(* Logix 5000 AddOnInstructionDefinition export Banner_VSM_Param_v4; software revision 33.00 *)

TYPE Banner_IOL_Port_v4 :   // UDT that has all of the data items necessary to communicate with a specific Port on a IO-Link Master
STRUCT
   Port_Controlled : INT;   // Each bit represents a port on an IO-Link Master. Set to 1 to tell AOI to control that port.
   Port_Activate : INT;   // Each bit represents a port on an IO-Link Master. When ON that port will process any commands in queue.
   Port_Read : INT;   // Each bit represents a port on an IO-Link Master. Used to determine when device AOI has requested a Read command.
   Port_Write : INT;   // Each bit represents a port on an IO-Link Master. Used to determine when device AOI has requested a Write command.
   Port_RW_Complete : INT;   // Each bit represents a port on an IO-Link Master. Tells device AOI that Read or Write request has been completed.
   Port_Device_Read : INT;
   Data_Transfer : SINT[190];   // Array to transfer data from IO-Master to device AOIs.
END_STRUCT
END_TYPE

TYPE Banner_VSM_RD_v4 :   // UDT that stores the Read Data for a VSM-2.
STRUCT
   Master_Cycle_Time : INT;
   Min_Cycle_Time : INT;
   Frame_Capability : INT;
   IO_Link_Version_ID : INT;
   Process_Data_Input_Length : INT;
   Process_Data_Output_Length : INT;
   Combined_Vendor_ID : DINT;   // IO-Link Vendor ID
   Vendor_ID1 : INT;
   Vendor_ID2 : INT;
   Combined_Device_ID : DINT;   // IO-Link Device ID
   Device_ID1 : INT;
   Device_ID2 : INT;
   Device_ID3 : INT;
   Maximum_Temp : INT;
   Actual_Temp : INT;
END_STRUCT
END_TYPE

TYPE Banner_VSM_v4 :   // All of the parameters for a VSM-2.
STRUCT
   Initial_Global_Read : BOOL;   // Determines if all of the IO-Link data has been read into the PLC yet
   Command : INT;   // Value placed in here will activate a read or write to a specifc IO-Link Index
   Read : Banner_VSM_RD_v4;   // Read Only Data
   Write : Banner_VSM_WD_v4;   // Write Data
   Archive : Banner_VSM_WD_v4;   // Archive Data
   Reset : BOOL;   // Resets AOI. This will force a complete parameter read of the sensor.
END_STRUCT
END_TYPE

TYPE Banner_VSM_WD_v4 :   // UDT that stores the Write Data for a VSM-2.
STRUCT
   Switching_Delay_TB : SINT;   // 0 = .1ms, 1 = .4ms, 2 = 1.6ms, 3 = 6.4ms.
   Output_Stretch_TB : SINT;   // 0 = .1ms, 1 = .4ms, 2 = 1.6ms, 3 = 6.4ms.
   Output_1_Config : SINT;   // 0 = Detection light on, 1 = Dection dark on, 2 = Stability alarm, 3 = Stability alarm inverted.
   Output_2_Config : SINT;   // 0 = Detection light on, 1 = Dection dark on, 2 = Stability alarm, 3 = Stability alarm inverted.
   Swtiching_Delay_Multiplier : INT;   // 0 to 255.
   Output_Stretch_Multiplier : INT;   // 0 to 255.
   Sensitivity : INT;   // 0 to 1023.
   Sequence_Choice : SINT;   // 0 to 9.
   Sensor_Mode : SINT;   // 1 = Fine, 2 = Normal, 3 = Fast.
   Teach_Command : SINT;   // 0 = Idle, 1 = Teach 1 Pt, 2 = Teach 2 Pt on target, 3 = Teach 2 Pt without target.
   Detection_Counter : DINT;   // 0 to 65535.
   Event_Flag_LED_Reg_Limit : SINT;
   Event_Flag_Disturbance_On_Receiver : SINT;
   Event_Flag_Under_Voltage_IOL : SINT;
   Event_Flag_Under_Voltage_Sensor : SINT;
   Event_Flag_Maximum_Temp : SINT;
   Event_Flag_EMC_Detected : SINT;
   Event_Flag_Short_Circuit_Detected : SINT;
END_STRUCT
END_TYPE

ADD_ON_INSTRUCTION Banner_VSM_Param_v4   (* revision 4.0, vendor Banner Engineering *)
// AOI to read and write parameter data to an IO-Link VSM-2.
VAR_IN_OUT
   VSM : Banner_VSM_v4; {required}
   Port_Data : Banner_IOL_Port_v4; {required}
END_VAR
VAR_INPUT
   Port : DINT; {required}
END_VAR
VAR
   Local_Control : DINT; {access None}
   Global_Read_Command_Value : INT; {access None}
   Global_Write_Command_Value : INT; {access None}
   Command_Being_Processed : BOOL; {access None}
   Update_Archive : BOOL; {access None}
   Index_Write_Inprocess : INT; {access None}
   Index_Write_Control : INT; {access None}
   Inprocess_Index : DINT; {access None}
END_VAR

ROUTINE Logic   (* ladder *)
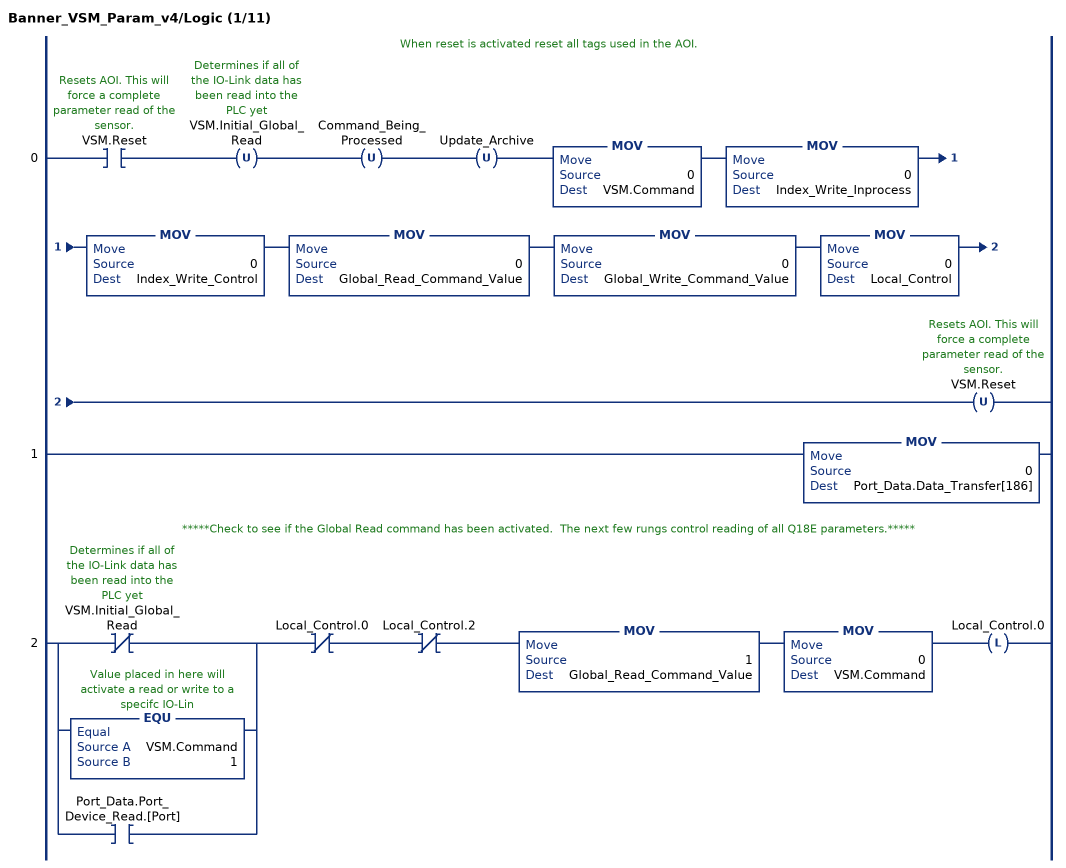
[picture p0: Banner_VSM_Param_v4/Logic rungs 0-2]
   // When reset is activated reset all tags used in the AOI.
   0: XIC(VSM.Reset)OTU(VSM.Initial_Global_Read)OTU(Command_Being_Processed)OTU(Update_Archive)MOV(0,VSM.Command)MOV(0,Index_Write_Inprocess)MOV(0,Index_Write_Control)MOV(0,Global_Read_Command_Value)MOV(0,Global_Write_Command_Value)MOV(0,Local_Control)OTU(VSM.Reset);
   1: MOV(0,Port_Data.Data_Transfer[186]);
   // *****Check to see if the Global Read command has been activated.  The next few rungs control reading of all Q18E parameters.*****
   2: [XIO(VSM.Initial_Global_Read) ,EQU(VSM.Command,1) ,XIC(Port_Data.Port_Device_Read.[Port]) ]XIO(Local_Control.0)XIO(Local_Control.2)MOV(1,Global_Read_Command_Value)MOV(0,VSM.Command)OTL(Local_Control.0);
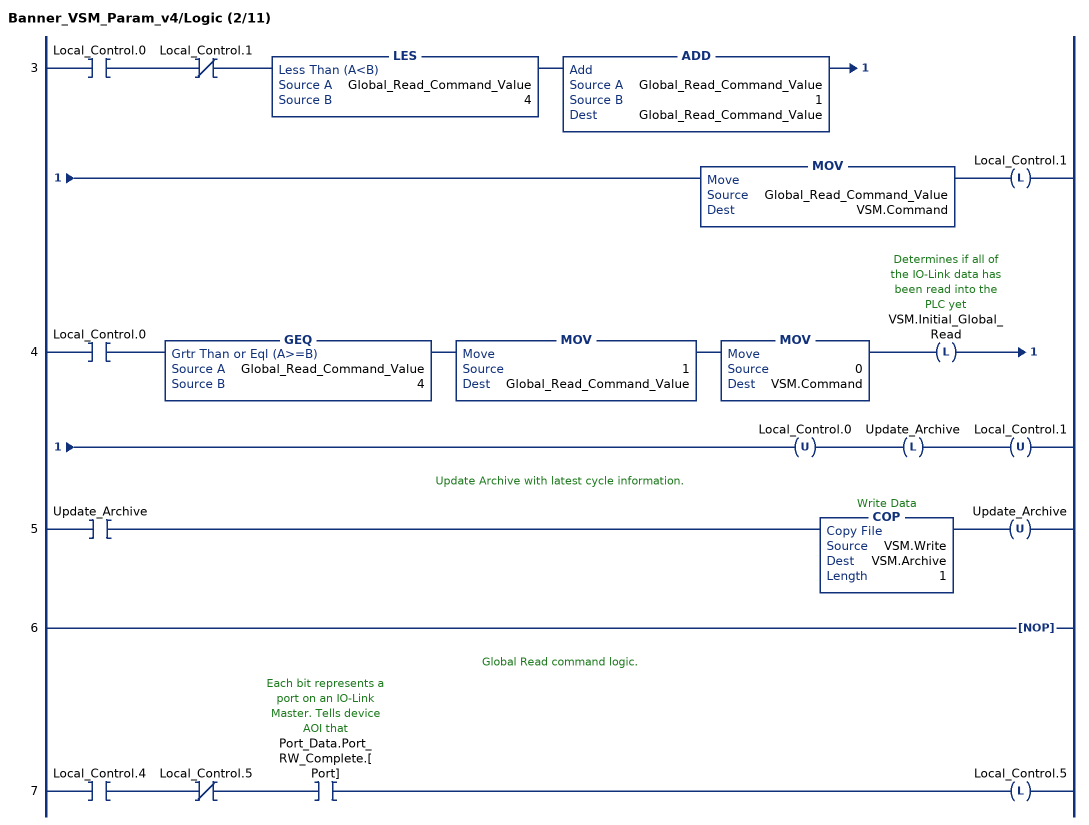
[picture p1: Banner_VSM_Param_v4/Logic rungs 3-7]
   3: XIC(Local_Control.0)XIO(Local_Control.1)LES(Global_Read_Command_Value,4)ADD(Global_Read_Command_Value,1,Global_Read_Command_Value)MOV(Global_Read_Command_Value,VSM.Command)OTL(Local_Control.1);
   4: XIC(Local_Control.0)GEQ(Global_Read_Command_Value,4)MOV(1,Global_Read_Command_Value)MOV(0,VSM.Command)OTL(VSM.Initial_Global_Read)OTU(Local_Control.0)OTL(Update_Archive)OTU(Local_Control.1);
   // Update Archive with latest cycle information.
   5: XIC(Update_Archive)COP(VSM.Write,VSM.Archive,1)OTU(Update_Archive);
   6: NOP();
   // Global Read command logic.
   7: XIC(Local_Control.4)XIO(Local_Control.5)XIC(Port_Data.Port_RW_Complete.[Port])OTL(Local_Control.5);
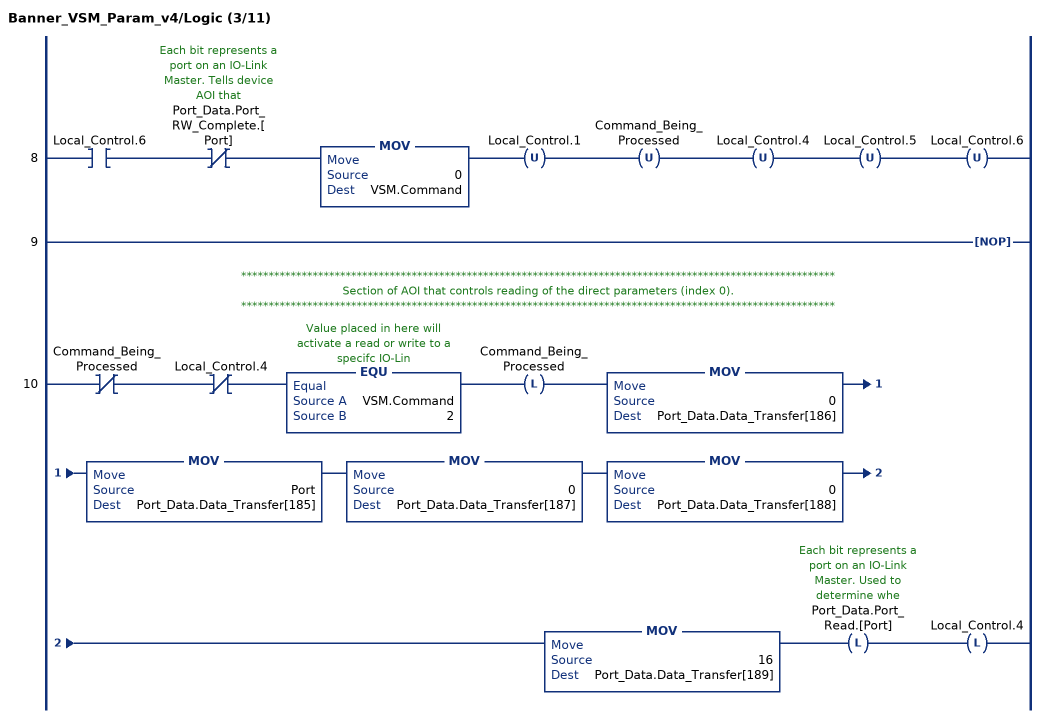
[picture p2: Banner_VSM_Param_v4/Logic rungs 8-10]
   8: XIC(Local_Control.6)XIO(Port_Data.Port_RW_Complete.[Port])MOV(0,VSM.Command)OTU(Local_Control.1)OTU(Command_Being_Processed)OTU(Local_Control.4)OTU(Local_Control.5)OTU(Local_Control.6);
   9: NOP();
   // ************************************************************************************************************
   // Section of AOI that controls reading of the direct parameters (index 0).
   // ************************************************************************************************************
   10: XIO(Command_Being_Processed)XIO(Local_Control.4)EQU(VSM.Command,2)OTL(Command_Being_Processed)MOV(0,Port_Data.Data_Transfer[186])MOV(Port,Port_Data.Data_Transfer[185])MOV(0,Port_Data.Data_Transfer[187])MOV(0,Port_Data.Data_Transfer[188])MOV(16,Port_Data.Data_Transfer[189])OTL(Port_Data.Port_Read.[Port])OTL(Local_Control.4);
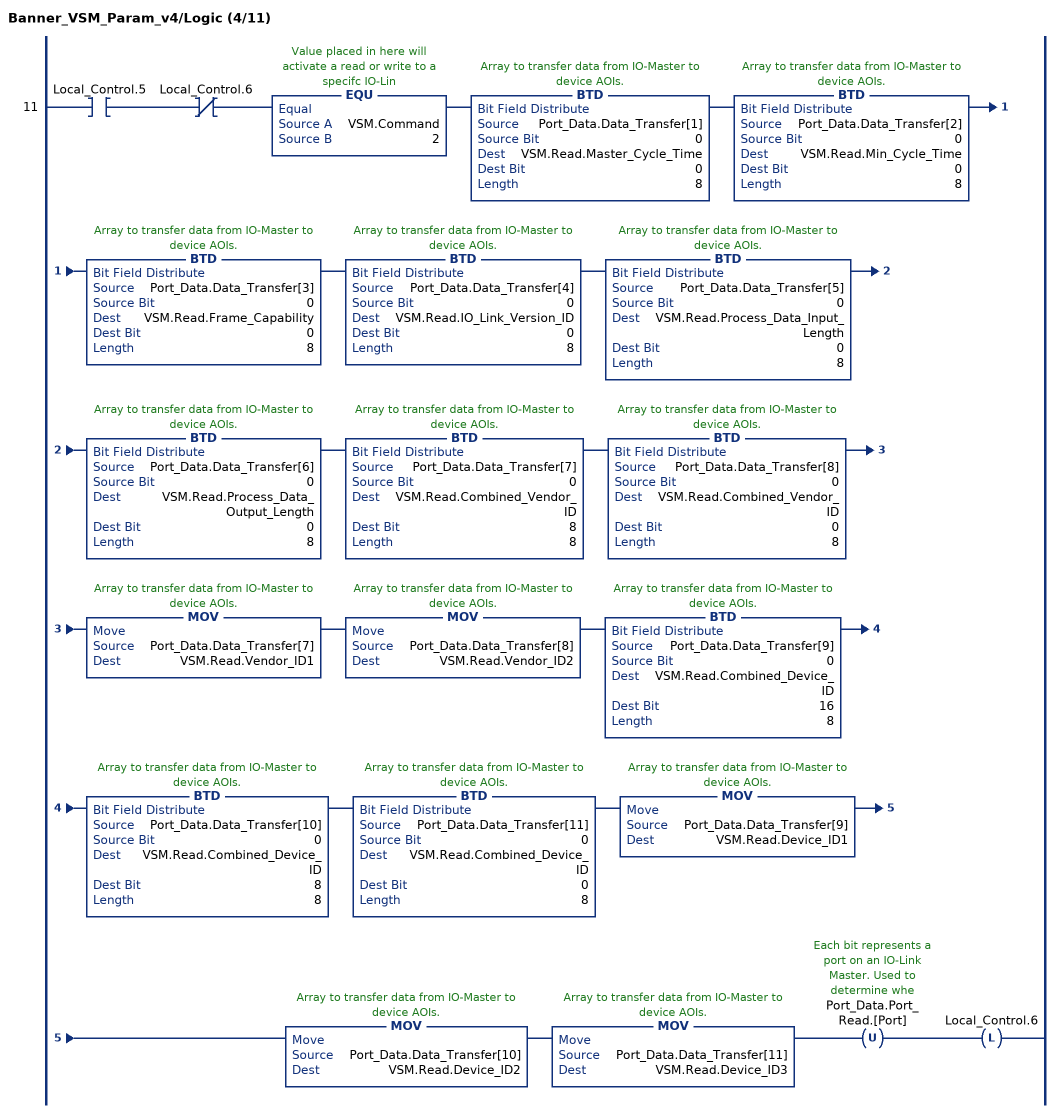
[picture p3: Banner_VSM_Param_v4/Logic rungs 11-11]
   11: XIC(Local_Control.5)XIO(Local_Control.6)EQU(VSM.Command,2)BTD(Port_Data.Data_Transfer[1],0,VSM.Read.Master_Cycle_Time,0,8)BTD(Port_Data.Data_Transfer[2],0,VSM.Read.Min_Cycle_Time,0,8)BTD(Port_Data.Data_Transfer[3],0,VSM.Read.Frame_Capability,0,8)BTD(Port_Data.Data_Transfer[4],0,VSM.Read.IO_Link_Version_ID,0,8)BTD(Port_Data.Data_Transfer[5],0,VSM.Read.Process_Data_Input_Length,0,8)BTD(Port_Data.Data_Transfer[6],0,VSM.Read.Process_Data_Output_Length,0,8)BTD(Port_Data.Data_Transfer[7],0,VSM.Read.Combined_Vendor_ID,8,8)BTD(Port_Data.Data_Transfer[8],0,VSM.Read.Combined_Vendor_ID,0,8)MOV(Port_Data.Data_Transfer[7],VSM.Read.Vendor_ID1)MOV(Port_Data.Data_Transfer[8],VSM.Read.Vendor_ID2)BTD(Port_Data.Data_Transfer[9],0,VSM.Read.Combined_Device_ID,16,8)BTD(Port_Data.Data_Transfer[10],0,VSM.Read.Combined_Device_ID,8,8)BTD(Port_Data.Data_Transfer[11],0,VSM.Read.Combined_Device_ID,0,8)MOV(Port_Data.Data_Transfer[9],VSM.Read.Device_ID1)MOV(Port_Data.Data_Transfer[10],VSM.Read.Device_ID2)MOV(Port_Data.Data_Transfer[11],VSM.Read.Device_ID3)OTU(Port_Data.Port_Read.[Port])OTL(Local_Control.6);
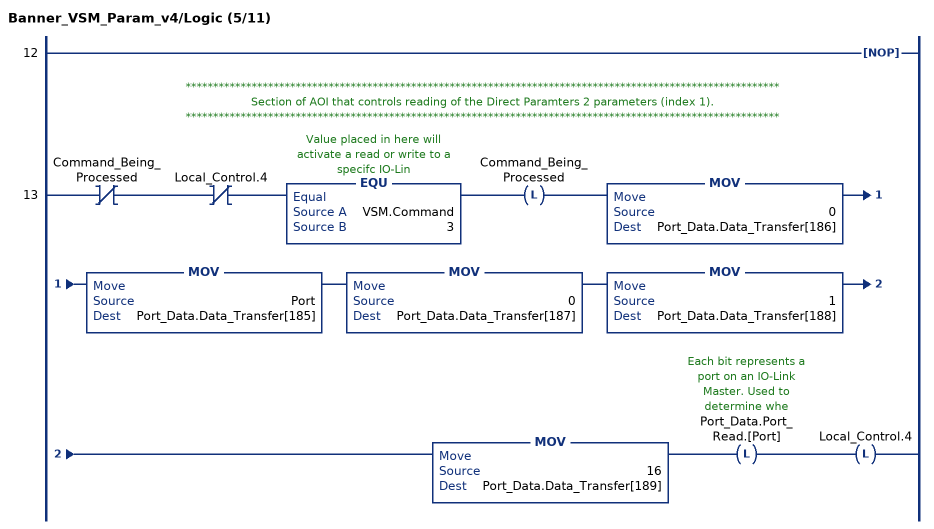
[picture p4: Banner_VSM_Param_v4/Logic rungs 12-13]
   12: NOP();
   // ************************************************************************************************************
   // Section of AOI that controls reading of the Direct Paramters 2 parameters (index 1).
   // ************************************************************************************************************
   13: XIO(Command_Being_Processed)XIO(Local_Control.4)EQU(VSM.Command,3)OTL(Command_Being_Processed)MOV(0,Port_Data.Data_Transfer[186])MOV(Port,Port_Data.Data_Transfer[185])MOV(0,Port_Data.Data_Transfer[187])MOV(1,Port_Data.Data_Transfer[188])MOV(16,Port_Data.Data_Transfer[189])OTL(Port_Data.Port_Read.[Port])OTL(Local_Control.4);
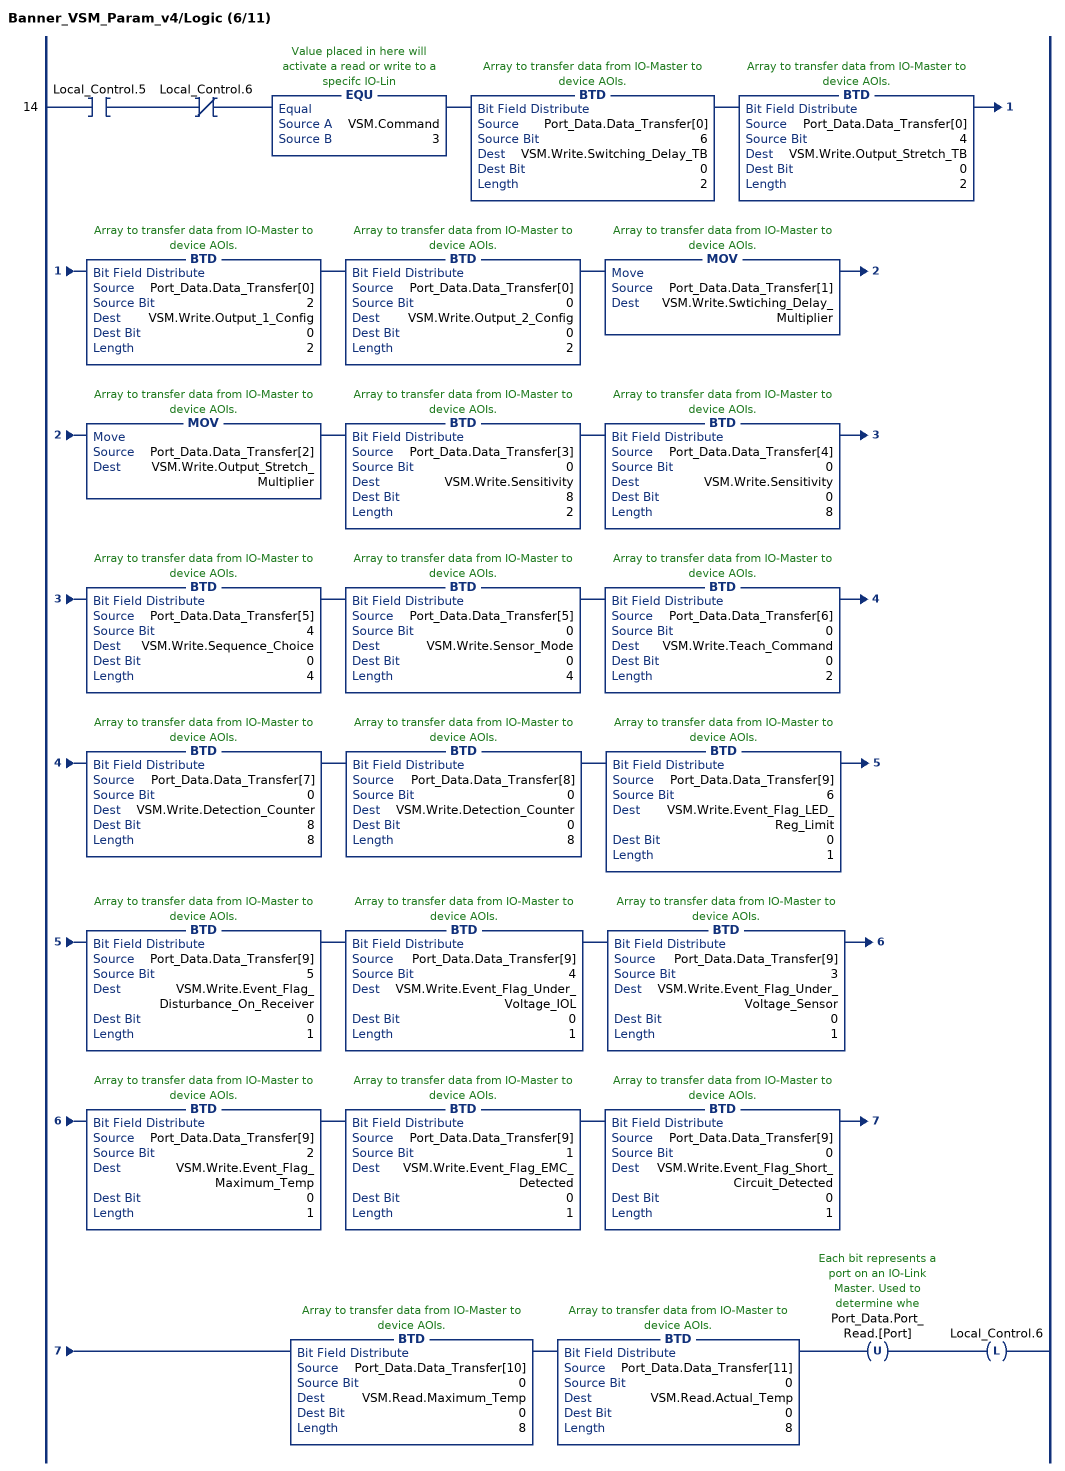
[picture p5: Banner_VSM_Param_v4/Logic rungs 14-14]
   14: XIC(Local_Control.5)XIO(Local_Control.6)EQU(VSM.Command,3)BTD(Port_Data.Data_Transfer[0],6,VSM.Write.Switching_Delay_TB,0,2)BTD(Port_Data.Data_Transfer[0],4,VSM.Write.Output_Stretch_TB,0,2)BTD(Port_Data.Data_Transfer[0],2,VSM.Write.Output_1_Config,0,2)BTD(Port_Data.Data_Transfer[0],0,VSM.Write.Output_2_Config,0,2)MOV(Port_Data.Data_Transfer[1],VSM.Write.Swtiching_Delay_Multiplier)MOV(Port_Data.Data_Transfer[2],VSM.Write.Output_Stretch_Multiplier)BTD(Port_Data.Data_Transfer[3],0,VSM.Write.Sensitivity,8,2)BTD(Port_Data.Data_Transfer[4],0,VSM.Write.Sensitivity,0,8)BTD(Port_Data.Data_Transfer[5],4,VSM.Write.Sequence_Choice,0,4)BTD(Port_Data.Data_Transfer[5],0,VSM.Write.Sensor_Mode,0,4)BTD(Port_Data.Data_Transfer[6],0,VSM.Write.Teach_Command,0,2)BTD(Port_Data.Data_Transfer[7],0,VSM.Write.Detection_Counter,8,8)BTD(Port_Data.Data_Transfer[8],0,VSM.Write.Detection_Counter,0,8)BTD(Port_Data.Data_Transfer[9],6,VSM.Write.Event_Flag_LED_Reg_Limit,0,1)BTD(Port_Data.Data_Transfer[9],5,VSM.Write.Event_Flag_Disturbance_On_Receiver,0,1)BTD(Port_Data.Data_Transfer[9],4,VSM.Write.Event_Flag_Under_Voltage_IOL,0,1)BTD(Port_Data.Data_Transfer[9],3,VSM.Write.Event_Flag_Under_Voltage_Sensor,0,1)BTD(Port_Data.Data_Transfer[9],2,VSM.Write.Event_Flag_Maximum_Temp,0,1)BTD(Port_Data.Data_Transfer[9],1,VSM.Write.Event_Flag_EMC_Detected,0,1)BTD(Port_Data.Data_Transfer[9],0,VSM.Write.Event_Flag_Short_Circuit_Detected,0,1)BTD(Port_Data.Data_Transfer[10],0,VSM.Read.Maximum_Temp,0,8)BTD(Port_Data.Data_Transfer[11],0,VSM.Read.Actual_Temp,0,8)OTU(Port_Data.Port_Read.[Port])OTL(Local_Control.6);
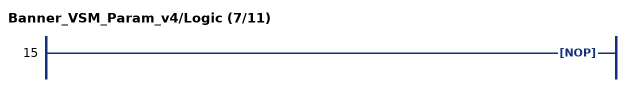
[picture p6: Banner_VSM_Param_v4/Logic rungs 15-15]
   15: NOP();
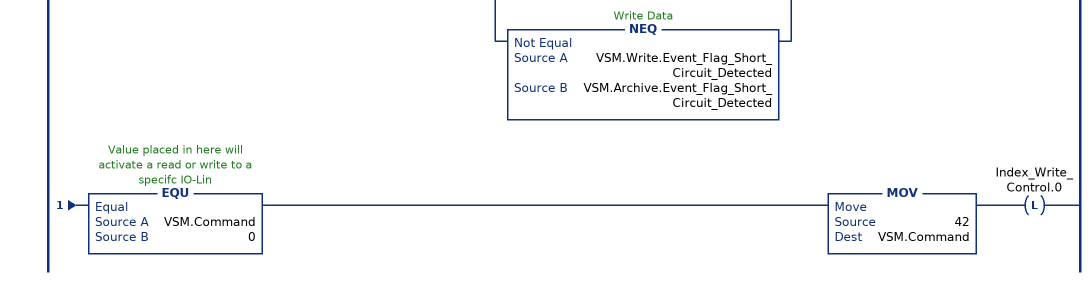
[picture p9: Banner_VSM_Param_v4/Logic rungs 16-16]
   // Check all Write parameters to see if they need to be updated.
   16: XIC(VSM.Initial_Global_Read)XIO(Local_Control.0)XIO(Index_Write_Control.0)XIO(Update_Archive)[NEQ(VSM.Write.Switching_Delay_TB,VSM.Archive.Switching_Delay_TB) ,NEQ(VSM.Write.Output_Stretch_TB,VSM.Archive.Output_Stretch_TB) ,NEQ(VSM.Write.Output_1_Config,VSM.Archive.Output_1_Config) ,NEQ(VSM.Write.Output_2_Config,VSM.Archive.Output_2_Config) ,NEQ(VSM.Write.Swtiching_Delay_Multiplier,VSM.Archive.Swtiching_Delay_Multiplier) ,NEQ(VSM.Write.Output_Stretch_Multiplier,VSM.Archive.Output_Stretch_Multiplier) ,NEQ(VSM.Write.Sensitivity,VSM.Archive.Sensitivity) ,NEQ(VSM.Write.Sequence_Choice,VSM.Archive.Sequence_Choice) ,NEQ(VSM.Write.Sensor_Mode,VSM.Archive.Sensor_Mode) ,NEQ(VSM.Write.Teach_Command,VSM.Archive.Teach_Command) ,NEQ(VSM.Write.Detection_Counter,VSM.Archive.Detection_Counter) ,NEQ(VSM.Write.Event_Flag_LED_Reg_Limit,VSM.Archive.Event_Flag_LED_Reg_Limit) ,NEQ(VSM.Write.Event_Flag_Disturbance_On_Receiver,VSM.Archive.Event_Flag_Disturbance_On_Receiver) ,NEQ(VSM.Write.Event_Flag_Under_Voltage_IOL,VSM.Archive.Event_Flag_Under_Voltage_IOL) ,NEQ(VSM.Write.Event_Flag_Under_Voltage_Sensor,VSM.Archive.Event_Flag_Under_Voltage_Sensor) ,NEQ(VSM.Write.Event_Flag_Maximum_Temp,VSM.Archive.Event_Flag_Maximum_Temp) ,NEQ(VSM.Write.Event_Flag_EMC_Detected,VSM.Archive.Event_Flag_EMC_Detected) ,NEQ(VSM.Write.Event_Flag_Short_Circuit_Detected,VSM.Archive.Event_Flag_Short_Circuit_Detected) ]OTL(Index_Write_Inprocess.0)XIO(Command_Being_Processed)EQU(VSM.Command,0)MOV(42,VSM.Command)OTL(Index_Write_Control.0);
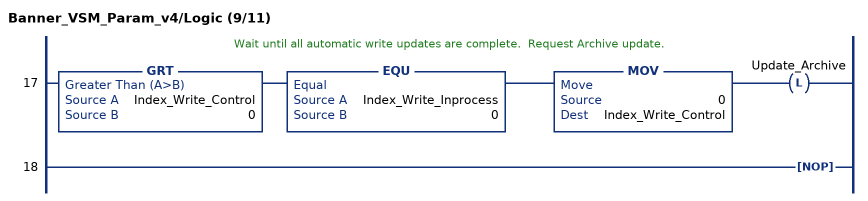
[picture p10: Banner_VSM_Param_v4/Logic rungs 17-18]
   // Wait until all automatic write updates are complete.  Request Archive update.
   17: GRT(Index_Write_Control,0)EQU(Index_Write_Inprocess,0)MOV(0,Index_Write_Control)OTL(Update_Archive);
   18: NOP();
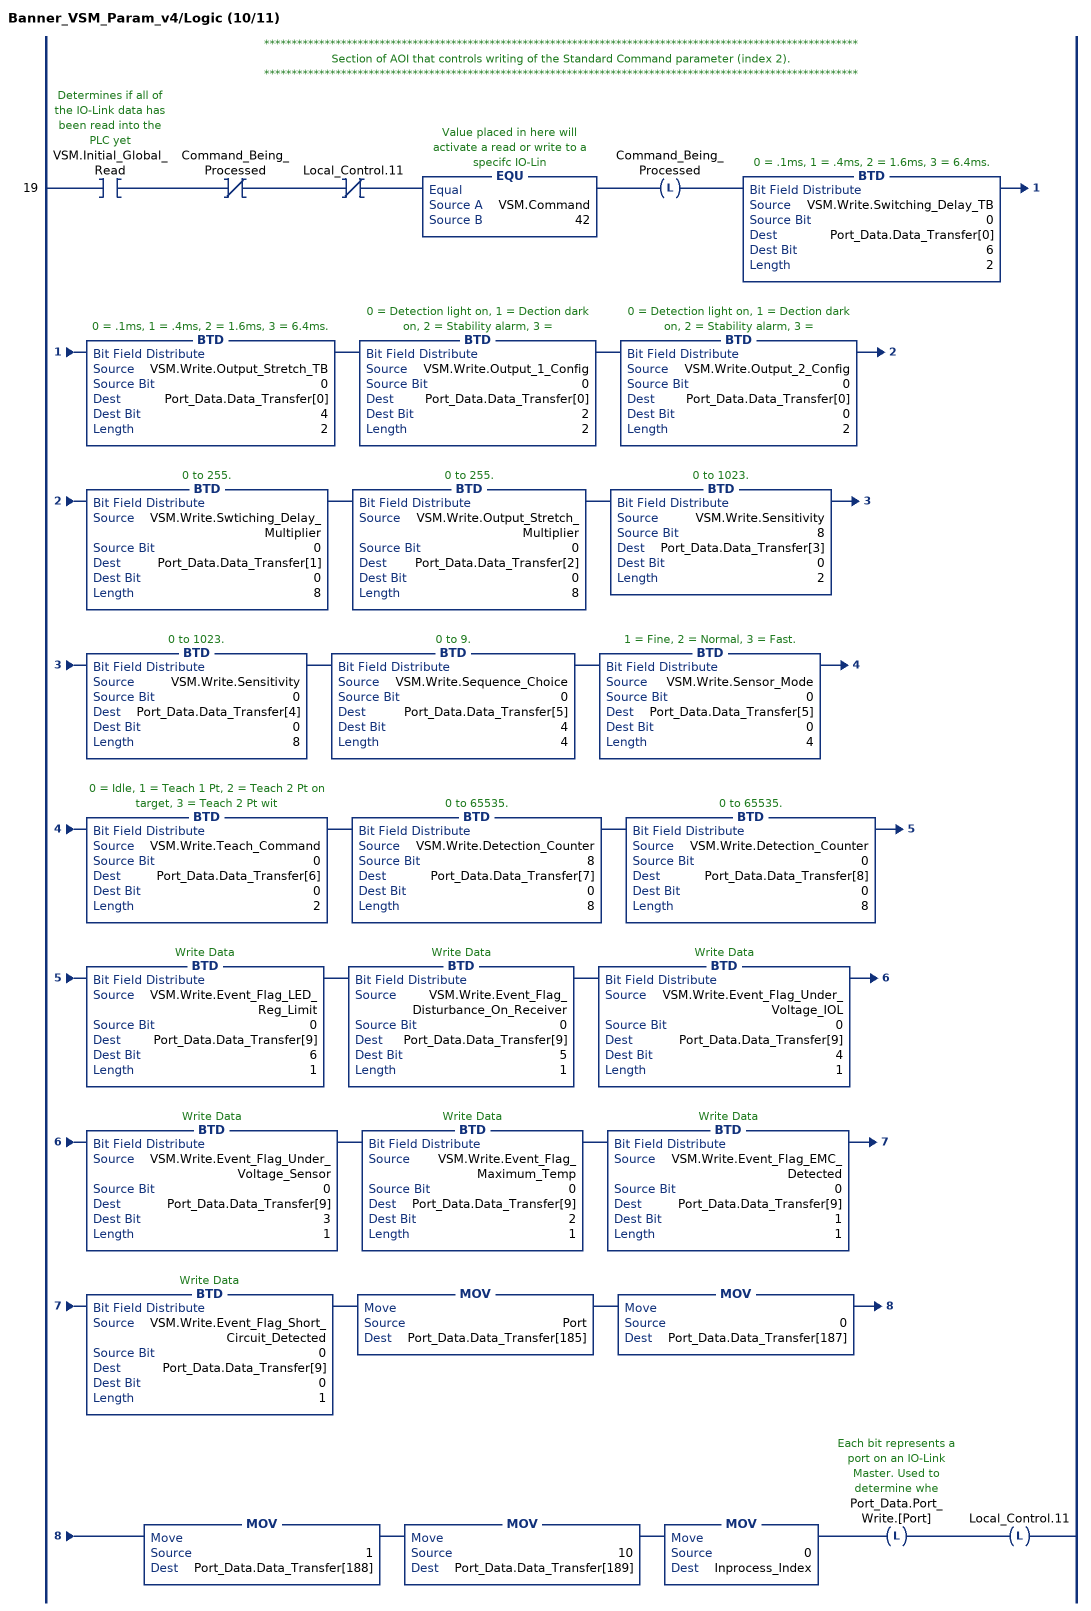
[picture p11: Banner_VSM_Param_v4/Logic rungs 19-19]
   // ************************************************************************************************************
   // Section of AOI that controls writing of the Standard Command parameter (index 2).
   // ************************************************************************************************************
   19: XIC(VSM.Initial_Global_Read)XIO(Command_Being_Processed)XIO(Local_Control.11)EQU(VSM.Command,42)OTL(Command_Being_Processed)BTD(VSM.Write.Switching_Delay_TB,0,Port_Data.Data_Transfer[0],6,2)BTD(VSM.Write.Output_Stretch_TB,0,Port_Data.Data_Transfer[0],4,2)BTD(VSM.Write.Output_1_Config,0,Port_Data.Data_Transfer[0],2,2)BTD(VSM.Write.Output_2_Config,0,Port_Data.Data_Transfer[0],0,2)BTD(VSM.Write.Swtiching_Delay_Multiplier,0,Port_Data.Data_Transfer[1],0,8)BTD(VSM.Write.Output_Stretch_Multiplier,0,Port_Data.Data_Transfer[2],0,8)BTD(VSM.Write.Sensitivity,8,Port_Data.Data_Transfer[3],0,2)BTD(VSM.Write.Sensitivity,0,Port_Data.Data_Transfer[4],0,8)BTD(VSM.Write.Sequence_Choice,0,Port_Data.Data_Transfer[5],4,4)BTD(VSM.Write.Sensor_Mode,0,Port_Data.Data_Transfer[5],0,4)BTD(VSM.Write.Teach_Command,0,Port_Data.Data_Transfer[6],0,2)BTD(VSM.Write.Detection_Counter,8,Port_Data.Data_Transfer[7],0,8)BTD(VSM.Write.Detection_Counter,0,Port_Data.Data_Transfer[8],0,8)BTD(VSM.Write.Event_Flag_LED_Reg_Limit,0,Port_Data.Data_Transfer[9],6,1)BTD(VSM.Write.Event_Flag_Disturbance_On_Receiver,0,Port_Data.Data_Transfer[9],5,1)BTD(VSM.Write.Event_Flag_Under_Voltage_IOL,0,Port_Data.Data_Transfer[9],4,1)BTD(VSM.Write.Event_Flag_Under_Voltage_Sensor,0,Port_Data.Data_Transfer[9],3,1)BTD(VSM.Write.Event_Flag_Maximum_Temp,0,Port_Data.Data_Transfer[9],2,1)BTD(VSM.Write.Event_Flag_EMC_Detected,0,Port_Data.Data_Transfer[9],1,1)BTD(VSM.Write.Event_Flag_Short_Circuit_Detected,0,Port_Data.Data_Transfer[9],0,1)MOV(Port,Port_Data.Data_Transfer[185])MOV(0,Port_Data.Data_Transfer[187])MOV(1,Port_Data.Data_Transfer[188])MOV(10,Port_Data.Data_Transfer[189])MOV(0,Inprocess_Index)OTL(Port_Data.Port_Write.[Port])OTL(Local_Control.11);
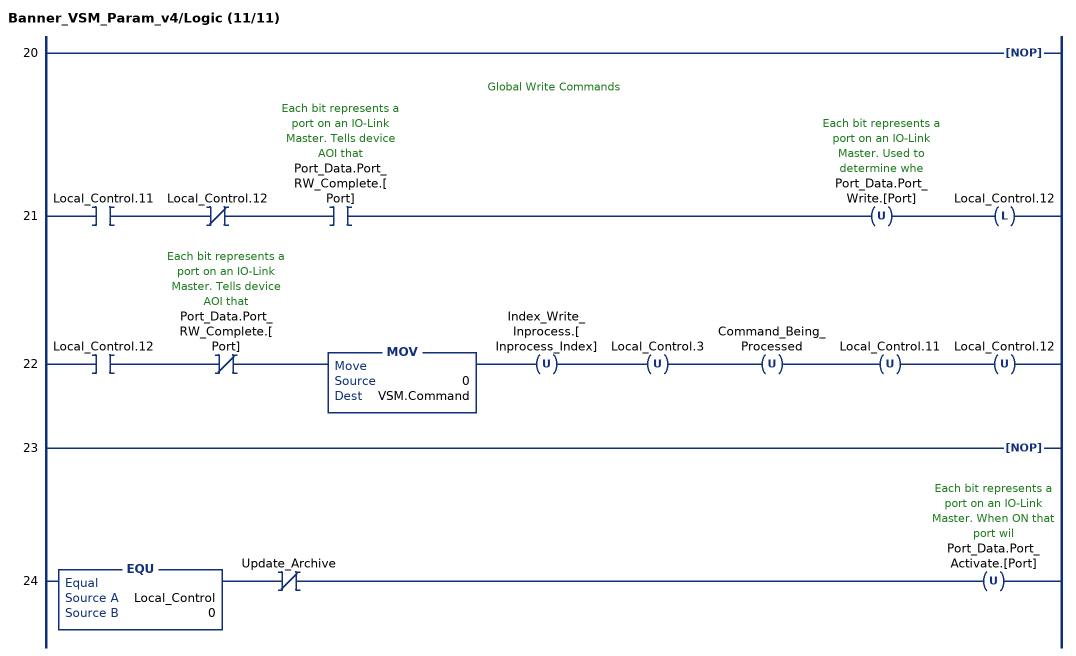
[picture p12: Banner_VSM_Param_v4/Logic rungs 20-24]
   20: NOP();
   // Global Write Commands
   21: XIC(Local_Control.11)XIO(Local_Control.12)XIC(Port_Data.Port_RW_Complete.[Port])OTU(Port_Data.Port_Write.[Port])OTL(Local_Control.12);
   22: XIC(Local_Control.12)XIO(Port_Data.Port_RW_Complete.[Port])MOV(0,VSM.Command)OTU(Index_Write_Inprocess.[Inprocess_Index])OTU(Local_Control.3)OTU(Command_Being_Processed)OTU(Local_Control.11)OTU(Local_Control.12);
   23: NOP();
   24: EQU(Local_Control,0)XIO(Update_Archive)OTU(Port_Data.Port_Activate.[Port]);
END_ROUTINE
END_ADD_ON_INSTRUCTION
